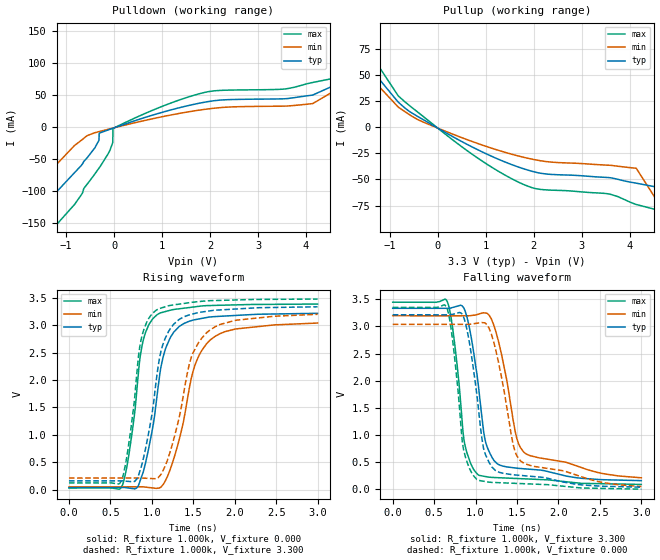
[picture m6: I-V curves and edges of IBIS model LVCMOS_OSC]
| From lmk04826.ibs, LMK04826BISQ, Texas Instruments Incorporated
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|   Model LVCMOS
[Model] LVCMOS_OSC
Model_type   Output
Polarity   Non-Inverting
Vmeas = 1.65
Vref = 1.65
Cref = 15pF
Rref = 50
|   typ   min   max
C_comp   2.0305p   1.9034p   2.088p
|   (nom PVT)   (slow PVT)   (fast PVT)
|C_comp (High state)   2.0305p   1.9034p   2.088p
|   (nom PVT)   (fast PVT)   (slow PVT)
|C_comp (Low state)   1.674p   1.576p   1.7125p
[Voltage Range]   3.3   3.15   3.45
[Temperature Range]   27   125   -40
[Pullup Reference]   3.3   3.15   3.45
[Pulldown Reference]   0   0   0
[Power Clamp Reference]   3.3   3.15   3.45
[GND Clamp Reference]   0   0   0
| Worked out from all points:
|   slope of the pulldown table from 0 to 0.495 V, typ, clamps not added: 39 ohm
|   slope of the pullup table from 0 to 0.495 V, typ, clamps not added: 39 ohm
|   falling waveform, R_fixture 1.000k, V_fixture 3.300: 20-80 % time 178ps typ, 232ps min, 140ps max; typ from 3.33 V to 0.161 V
|   rising waveform, R_fixture 1.000k, V_fixture 0.000: 20-80 % time 217ps typ, 286ps min, 165ps max; typ from 0.04 V to 3.22 V
|   rising waveform, R_fixture 1.000k, V_fixture 3.300: 20-80 % time 216ps typ, 290ps min, 164ps max; typ from 0.161 V to 3.33 V
|   falling waveform, R_fixture 1.000k, V_fixture 0.000: 20-80 % time 173ps typ, 228ps min, 136ps max; typ from 3.22 V to 0.04 V
[Pulldown]
|   Voltage   I(typ)   I(min)   I(max)
-3.3V     -785.5mA   -668.8mA   -867.2mA
-2.023V   -246.5mA   -189mA     -294.6mA
-1.795V   -190.1mA   -138.6mA   -222.1mA
-1.384V   -116.4mA   -73.03mA   -168.4mA
-270.6mV  -8.334mA   -6.174mA   -59.44mA
-28.05mV  -1.86mA    -1.561mA   -24.12mA
-23.1mV   -1.728mA   -1.467mA   -2.069mA
1.883V    39.05mA    27.81mA    54.38mA
4.14V     50.34mA    36.91mA    70.06mA
4.882V    75.33mA    69.76mA    81.21mA
5.857V    139.3mA    152.4mA    153.1mA
6.595V    236.7mA    234.9mA    258.1mA
[Pullup]
|   Voltage   I(typ)   I(min)   I(max)
-3.3V     231.3mA    210.5mA    276.4mA
-2.439V   117.7mA    114.3mA    148.6mA
-2.117V   95.35mA    82.53mA    119.7mA
-597.3mV  15.15mA    12.07mA    20.85mA
1.808V    -40.09mA   -29.02mA   -55.2mA
3.551V    -48.13mA   -36.34mA   -63.71mA
4.135V    -53.52mA   -39.28mA   -73.88mA
4.531V    -56.99mA   -67.68mA   -78.6mA
4.536V    -92.41mA   -68.19mA   -78.65mA
4.848V    -132.4mA   -102.4mA   -82.42mA
4.853V    -133.1mA   -103mA     -162.6mA
6.595V    -760.8mA   -664.5mA   -800.4mA
[Ramp]
R_load = 1000
|   typ   min   max
dV/dt_r   1.90033/2.16555e-10   1.77642/2.86485e-10   2.00968/1.6517e-10
dV/dt_f   1.9019/1.78168e-10   1.76631/2.32547e-10   2.01351/1.3979e-10
[Falling Waveform]
R_fixture = 1.000k
V_fixture = 3.300
V_fixture_min = 3.150
V_fixture_max = 3.450
C_fixture = 0.000
|  time   V(typ)   V(min)   V(max)
0s        3.335V     3.198V     3.447V
658.8ps   3.335V     3.197V     3.458V
748.1ps   3.361V     3.197V     2.679V
862.4ps   3.326V     3.197V     892.9mV
1.033ns   1.92V      3.227V     267.3mV
1.111ns   940.9mV    3.249V     239mV
1.198ns   589.5mV    3.109V     220.4mV
1.497ns   390.3mV    941.2mV    200.2mV
1.581ns   379.6mV    687.2mV    194.6mV
3ns       160.7mV    212.9mV    90.81mV
[Rising Waveform]
R_fixture = 1.000k
V_fixture = 0.000
V_fixture_min = 0.000
V_fixture_max = 0.000
C_fixture = 0.000
|  time   V(typ)   V(min)   V(max)
0s        40.31mV    52.07mV    31.96mV
644.8ps   40.69mV    52.44mV    80mV
759.4ps   22.69mV    52.5mV     1.012V
884.1ps   270.9mV    52.57mV    2.643V
1.062ns   1.702V     25.8mV     3.188V
1.14ns    2.441V     101.5mV    3.239V
1.264ns   2.873V     564.1mV    3.286V
1.497ns   3.092V     2.158V     3.33V
1.672ns   3.143V     2.68V      3.357V
3ns       3.216V     3.039V     3.385V
[Rising Waveform]
R_fixture = 1.000k
V_fixture = 3.300
V_fixture_min = 3.150
V_fixture_max = 3.450
C_fixture = 0.000
|  time   V(typ)   V(min)   V(max)
0s        160.7mV    212.9mV    123.4mV
632.9ps   161.5mV    213.4mV    160.4mV
737.4ps   149.1mV    213.5mV    999.6mV
868.3ps   399.5mV    213.6mV    2.72V
1.05ns    1.959V     205.9mV    3.27V
1.121ns   2.587V     307mV      3.316V
1.222ns   2.934V     697mV      3.36V
1.476ns   3.197V     2.413V     3.415V
1.66ns    3.252V     2.86V      3.443V
3ns       3.335V     3.198V     3.476V
[Falling Waveform]
R_fixture = 1.000k
V_fixture = 0.000
V_fixture_min = 0.000
V_fixture_max = 0.000
C_fixture = 0.000
|  time   V(typ)   V(min)   V(max)
0s        3.216V     3.039V     3.352V
644.8ps   3.215V     3.039V     3.375V
727.9ps   3.225V     3.039V     2.684V
849.8ps   3.189V     3.039V     774.3mV
1.016ns   1.736V     3.06V      180.9mV
1.095ns   763.1mV    3.069V     150.4mV
1.166ns   488.6mV    2.955V     132.2mV
1.451ns   269.1mV    839.8mV    112.5mV
1.547ns   256.4mV    517.3mV    106.5mV
3ns       40.31mV    52.07mV    3.732mV
